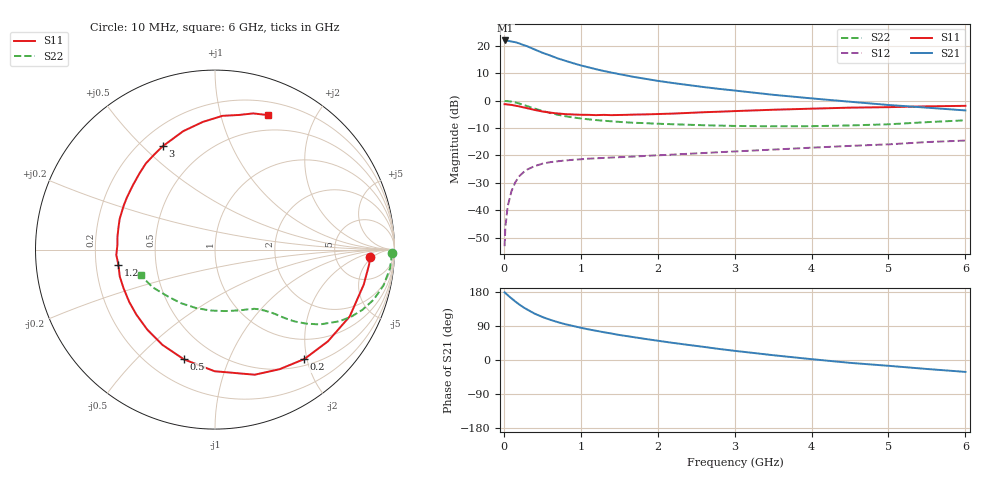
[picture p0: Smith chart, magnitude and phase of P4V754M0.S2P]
! SIEMENS Small Signal Semiconductors
! BFP182
! Si NPN RF Bipolar Junction Transistor in SOT143
! VCE = 0.75 V  IC = 4 mA
! Common Emitter S-Parameters:  March  1996
# GHz  S  MA  R  50
!  f  S11  S21  S12  S22
! GHz  MAG  ANG  MAG  ANG  MAG  ANG  MAG  ANG
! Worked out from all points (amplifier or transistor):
!   36 points, 10 MHz to 6 GHz, reference 50 ohm
!   highest |S21| = 22.0 dB at 20 MHz (marker M1)
!   |S21| within 3 dB of that: start of sweep to 376.3 MHz
!   unconditionally stable (mu >= 1): 1.571 GHz to end of sweep
!   at 250 MHz: K = 0.20, MSG = 23.3 dB, |S12| = -26.3 dB
!   at 1.4 GHz: K = 0.92, MSG = 15.5 dB, |S12| = -20.8 dB
!   at 6 GHz: K = 1.08, MAG = 3.8 dB, |S12| = -14.6 dB
!   S11 on the Smith chart (normalised r, x): 10 MHz: 12, -4; 200 MHz: 0.61, -1.95; 500 MHz: 0.34, -0.70; 1.2 GHz: 0.30, -0.07; 3 GHz: 0.29, +0.58; 6 GHz: 0.33, +1.42
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0.01  0.8625 -2.7  12.41 178.5  0.0022 80.9  0.9887 -1.2
0.02  0.863 -5.4  12.6 177.0  0.0049 89.1  0.9844 -2.4
0.05  0.8514 -13.2  12.46 171.1  0.0117 84.8  0.981 -6.1
0.1  0.8379 -26.4  12.04 162.6  0.0224 75.4  0.9599 -12.0
0.15  0.8105 -39.1  11.7 154.2  0.0325 68.4  0.9269 -17.5
0.2  0.7871 -50.8  11.13 146.6  0.0417 63.8  0.8876 -22.2
0.25  0.7571 -61.7  10.45 139.6  0.0485 57.8  0.8443 -26.4
0.3  0.7313 -72.4  9.909 133.6  0.0549 53.4  0.7989 -30.0
0.4  0.6776 -90.2  8.632 122.4  0.0638 46.1  0.718 -35.5
0.5  0.6356 -105.8  7.525 113.6  0.0706 40.6  0.652 -39.2
0.6  0.6062 -118.9  6.708 106.3  0.0753 36.6  0.5987 -42.0
0.7  0.584 -130.3  5.926 100.0  0.0782 33.6  0.5547 -44.0
0.8  0.5684 -140.4  5.358 94.4  0.0808 31.2  0.5205 -45.6
1.1  0.5513 -164.3  4.073 80.8  0.0872 26.9  0.4566 -49.3
1.2  0.5448 -170.9  3.754 77.1  0.0886 25.9  0.4422 -50.5
1.7  0.5578 162.3  2.702 59.9  0.0955 24.4  0.3942 -56.8
2.2  0.5813 141.9  2.1 45.1  0.1036 23.6  0.3713 -64.9
3  0.6454 116.8  1.532 24.2  0.1182 21.9  0.3458 -81.9
3.5  0.6833 105.0  1.282 12.7  0.1279 20.2  0.3403 -94.6
4.5  0.7464 86.8  0.957 -7.5  0.1493 16.1  0.3533 -122.3
5.5  0.7882 74.3  0.746 -23.7  0.1755 11.3  0.4055 -148.7
6  0.8053 68.5  0.664 -31.4  0.1869 7.3  0.438 -160.8
